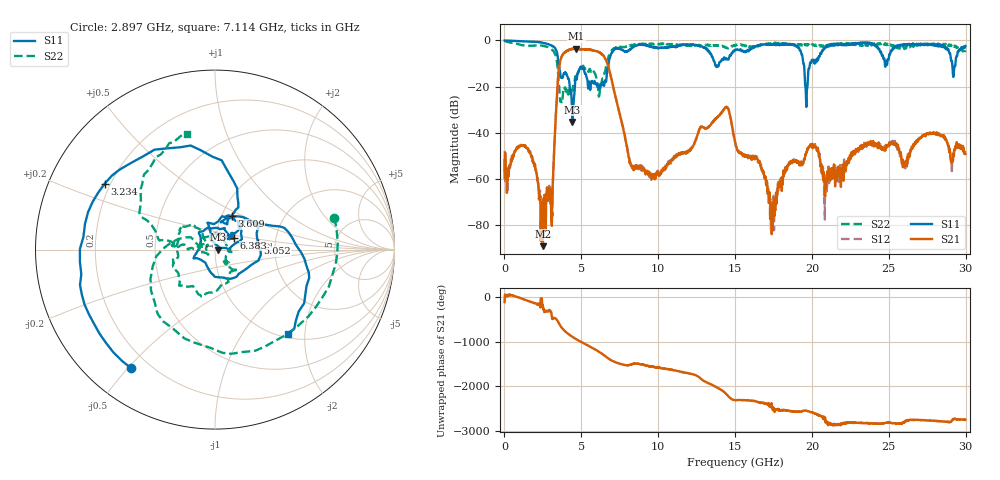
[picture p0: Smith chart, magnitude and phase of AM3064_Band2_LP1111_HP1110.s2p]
# Hz S DB R 50.0
!freq dBS11 angS11 dBS21 angS21 dBS12 angS12 dBS22 angS22
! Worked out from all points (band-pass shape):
!   1600 points, 10 MHz to 29.98 GHz, reference 50 ohm
!   highest |S21| = -3.54 dB at 4.677 GHz (marker M1); lowest = -88.9 dB at 2.503 GHz (marker M2)
!   |S21| within 3 dB of the highest: 3.758 GHz to 6.426 GHz (2.668 GHz wide, 52.4 % of centre)
!   lowest |S11| = -35.3 dB at 4.415 GHz (marker M3), VSWR 1.04, Z = 51.8 + j0.011 ohm
!   |S11| at or under -10 dB: 3.518 GHz to 6.778 GHz (3.26 GHz wide, 63.3 % of centre); 13.69 GHz to 13.96 GHz (271.9 MHz wide, 1.97 % of centre); 19.44 GHz to 19.88 GHz (432.9 MHz wide, 2.2 % of centre)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
!   |S22| runs from -26.8 to -0.1 dB; largest |S21 - S12| = 0.016
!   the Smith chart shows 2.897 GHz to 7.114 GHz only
!   S11 on the Smith chart (normalised r, x): 2.897 GHz: 0.13, -0.51; 3.234 GHz: 0.18, +0.27; 3.609 GHz: 1.11, +0.44; 5.052 GHz: 1.62, +0.13; 6.383 GHz: 1.22, +0.17; 7.114 GHz: 1.08, -1.64
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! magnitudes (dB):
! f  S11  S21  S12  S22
! 10 MHz  -0.1  -51.6  -47.7  -0.1
! 1.416 GHz  -0.5  -46.1  -46.0  -2.4
! 2.503 GHz  -1.1  -88.9  -70.0  -2.5
! 2.897 GHz  -1.8  -66.5  -64.1  -3.2
! 3.234 GHz  -2.9  -47.4  -47.9  -5.2
! 3.609 GHz  -13.6  -9.7  -9.5  -25.2
! 4.415 GHz  -35.3  -3.8  -3.7  -21.4
! 4.677 GHz  -16.6  -3.5  -3.5  -16.4
! 5.015 GHz  -12.1  -3.8  -3.8  -12.0
! 5.052 GHz  -12.3  -3.9  -3.8  -11.9
! 6.383 GHz  -18.1  -6.3  -6.4  -16.4
! 7.114 GHz  -4.2  -21.3  -21.4  -3.6
! 8.276 GHz  -3.1  -54.0  -54.6  -2.1
! 10 GHz  -3.3  -57.5  -57.2  -1.7
! 14.39 GHz  -8.2  -29.0  -29.0  -3.2
! 15 GHz  -4.0  -44.5  -44.1  -2.1
! 17.46 GHz  -1.6  -70.4  -78.0  -1.4
! 19.65 GHz  -24.1  -48.4  -48.3  -1.7
! 19.99 GHz  -8.5  -45.2  -45.4  -1.7
! 20.91 GHz  -2.6  -64.3  -61.0  -2.6
! 25 GHz  -8.0  -45.1  -44.7  -1.6
! 29.98 GHz  -2.4  -49.1  -49.3  -4.3
